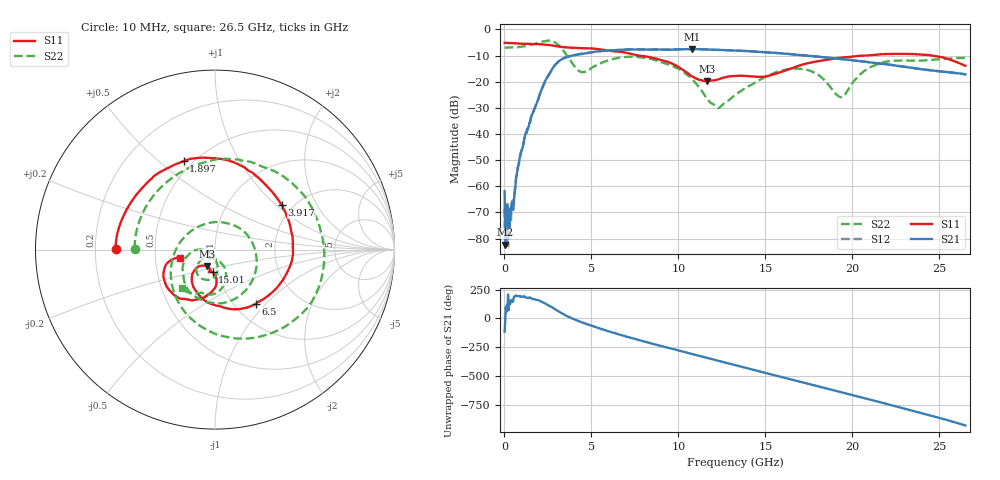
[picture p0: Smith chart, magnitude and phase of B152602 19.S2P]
!  2-Port S-parameters saved by WinCal
! VAR MeasName=S-Parameters (CALIBRATED_DATA) read from VNA (N5242A)
! VAR MeasDate=2016-1-5 16:28:07
! VAR NAME=B152602 19
! VAR FILENAME=B152602 19.S2P
! VAR DATE=2016-1-5 16:28:07
! VAR PHYS_PORTS=1,2
# Hz S DB R 50
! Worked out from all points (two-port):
!   801 points, 10 MHz to 26.5 GHz, reference 50 ohm
!   highest |S21| = -7.52 dB at 10.8 GHz (marker M1); lowest = -82.3 dB at 43.11 MHz (marker M2)
!   |S21| within 3 dB of the highest: 3.606 GHz to 18.17 GHz (14.56 GHz wide, 134 % of centre)
!   lowest |S11| = -19.7 dB at 11.63 GHz (marker M3), VSWR 1.23, Z = 44.9 - j8.5 ohm
!   |S11| at or under -10 dB: 7.72 GHz to 20.7 GHz (12.98 GHz wide, 91.3 % of centre); 24.62 GHz to end of sweep
!   |S22| runs from -30.1 to -4.2 dB; largest |S21 - S12| = 0.003
!   S11 on the Smith chart (normalised r, x): 10 MHz: 0.29, +0.00; 1.897 GHz: 0.45, +0.61; 3.917 GHz: 1.75, +1.09; 6.5 GHz: 1.24, -0.88; 15.01 GHz: 0.94, -0.24; 26.5 GHz: 0.67, -0.06
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1e7  -5.13 179.6  -61.93 -115.4  -68.59 -11.4  -6.96 179.4
4.31125e7  -5.13 178.3  -82.34 -29.6  -81.86 83.4  -6.97 177.4
1.755625e8  -5.15 173.0  -67.66 77.9  -66.29 87.7  -6.95 169.2
3.41125e8  -5.21 166.6  -68.37 135.3  -70.75 114.8  -6.93 159.0
1.003375e9  -5.47 142.5  -46.07 -171.2  -46.05 -172.1  -6.60 117.5
1.897412e9  -5.63 109.5  -27.47 159.8  -27.46 159.9  -5.21 52.6
2.493438e9  -5.92 85.6  -17.97 116.2  -17.97 116.1  -4.28 -4.9
2.990125e9  -6.44 66.2  -13.03 72.8  -13.04 72.7  -5.35 -65.2
3.4537e9  -6.83 49.9  -10.90 31.8  -10.91 31.8  -8.70 -121.5
3.917275e9  -7.00 33.7  -9.97 -1.7  -9.97 -1.6  -13.10 -178.1
4.447075e9  -7.19 14.8  -9.35 -33.9  -9.34 -33.8  -16.34 107.2
6.50005e9  -8.46 -53.2  -7.89 -135.1  -7.87 -135.1  -10.93 -53.0
8.851038e9  -11.44 -109.5  -7.69 126.1  -7.65 126.0  -12.21 -134.3
1.080468e10  -18.04 -132.8  -7.52 50.4  -7.51 50.3  -19.04 -178.2
1.163249e10  -19.66 -115.8  -7.67 17.2  -7.66 17.3  -26.36 -171.7
1.229474e10  -19.11 -104.5  -7.81 -8.3  -7.80 -8.2  -30.13 -129.0
1.3255e10  -17.84 -104.4  -8.08 -45.5  -8.07 -45.6  -25.08 -88.4
1.500996e10  -17.96 -95.9  -8.72 -113.6  -8.72 -113.9  -18.12 -84.4
1.769208e10  -12.56 -94.4  -10.23 142.4  -10.18 142.5  -16.15 -131.8
1.938081e10  -10.78 -107.5  -11.36 77.7  -11.35 77.5  -25.95 -97.5
2.209604e10  -9.38 -130.1  -13.48 -28.6  -13.42 -29.0  -12.17 -90.7
2.65e10  -13.91 -167.1  -17.18 149.0  -17.18 148.9  -10.97 -130.4
